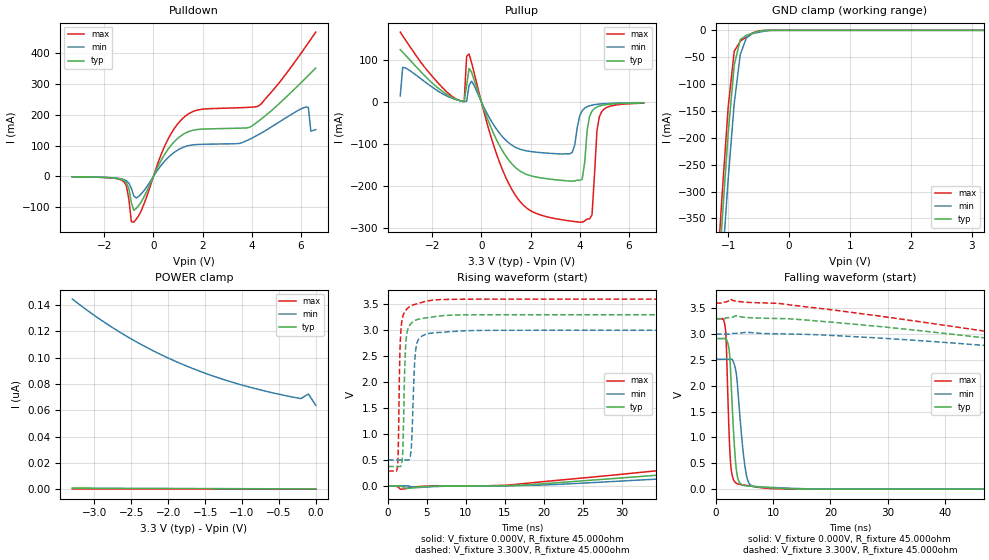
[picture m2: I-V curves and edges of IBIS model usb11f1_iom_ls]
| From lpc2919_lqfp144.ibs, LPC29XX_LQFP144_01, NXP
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| usb11f1
|   Universal Serial Bus Pad
|   Revision 1.1 Specification
|   Programmable Single Ended Core Input
|   Forced Single Ended Low
|   Switchable between
|   - high speed output mode
|   - low speed output mode
|   - low/high speed input mode
| |   Rev 0.20 IBIS Model Design Automation Generation   |
| |   N O N - S I L I C O N   C O R R E L A T E D   |
| |   This IBIS [Model] is pre-Beta tactical support   |
| |  Note: this IBIS [Model] contains clamp curves generated   |
| |   through simulation which should not be relied upon   |
| Pccmos14 hliolib_nlm 4.0
|   0.18 um 3.3V pad library
|   six level metal
|   dual oxide
|   single threshold voltage
|   nominal line mixed supply
|   parasitic extracted netlists
| Process block c14
| Low Speed Output Mode
[Model]   usb11f1_iom_ls | of usb11f1
Model_type   I/O
Polarity   Non-Inverting
Enable   Active-Low
|  Reciever Thresholds
Vinl   = 0.8V
Vinh   = 2.0V
| AC Test Load Conditions
Vref   = 0
Cref   = 0
Rref   = 1000000000
Vmeas   = 1.65
| [Process Range]   typical   min   max
| C_comp edge width   400.000ps   400.000ps   400.000ps
| C_comp Tstrobe   40.000fs   40.000fs   40.000fs
C_comp   3.752pF   3.496pF   4.045pF
[Temperature Range]   25   125   -40
[Voltage Range]   3.30V   3.00V   3.60V
[GND Clamp Reference]   0.00V   0.00V   0.00V
[Pulldown Reference]   0.00V   0.00V   0.00V
[POWER Clamp Reference]   3.30V   3.00V   3.60V
[Pullup Reference]   3.30V   3.00V   3.60V
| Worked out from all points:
|   slope of the pulldown table from 0 to 0.495 V, typ, clamps not added: 6.48 ohm
|   slope of the pullup table from 0 to 0.495 V, typ, clamps not added: 6.61 ohm
|   GND clamp passes 1 mA (typ) near -0.46 V on its own axis
|   rising waveform, V_fixture 0.000V, R_fixture 45.000ohm: 20-80 % time 151ns typ, 180ns min, 132ns max; typ from 0 V to 2.91 V
|   falling waveform, V_fixture 0.000V, R_fixture 45.000ohm: 20-80 % time 850ps typ, 1.23ns min, 609ps max; typ from 2.91 V to 0 V
|   rising waveform, V_fixture 3.300V, R_fixture 45.000ohm: 20-80 % time 318ps typ, 398ps min, 284ps max; typ from 0.374 V to 3.3 V
|   falling waveform, V_fixture 3.300V, R_fixture 45.000ohm: 20-80 % time 156ns typ, 194ns min, 133ns max; typ from 3.3 V to 0.38 V
[GND Clamp]
| ref voltage   0.00V   0.00V   0.00V
|   Voltage   I(typ)   I(min)   I(max)
-3.3V     -4.618A    -4.67A     -4.591A
-1.2V     -533.4mA   -616mA     -486.2mA
-1.1V     -356.1mA   -441.1mA   -306.9mA
-1V       -192.1mA   -277.1mA   -143.8mA
-900mV    -64.59mA   -135.6mA   -38.91mA
-800mV    -17.04mA   -44.51mA   -19.95mA
-700mV    -9.237mA   -13.86mA   -12.52mA
-600mV    -5.456mA   -6.064mA   -4.789mA
-500mV    -1.495mA   -3.666mA   -840.2uA
-300mV    -6.625uA   -179.7uA   -408.9nA
3.2V      293.2pA    68.89nA    105.6pA
[Power Clamp]   | Vtable = Vcc - Vpad
| ref voltage   3.30V   3.00V   3.60V
|   Voltage   I(typ)   I(min)   I(max)
-3.3V     1.005nA    144.5nA    354.7pA
-3V       911.2pA    132nA      335.1pA
-2.6V     800.8pA    117.4nA    309pA
-2.3V     727.5pA    108nA      289.6pA
-1.9V     640.7pA    97.15nA    263.8pA
-1.6V     582.9pA    90.25nA    244.5pA
-1.3V     530.6pA    84.3nA     225.3pA
-1V       483pA      79.18nA    206.1pA
-700mV    439.6pA    74.79nA    187pA
-200mV    377.6pA    68.89nA    155pA
-100mV    416.5pA    72.39nA    142.6pA
0V        319.1pA    63.83nA    125.6pA
[Pulldown]
| ref voltage   0.00V   0.00V   0.00V
|   Voltage   I(typ)   I(min)   I(max)
-3.3V     -1.652mA   -1.454mA   -1.796mA
-1.2V     -13.92mA   -10.45mA   -17.73mA
-1.1V     -21.12mA   -14.45mA   -30.61mA
-900mV    -85.23mA   -38.63mA   -146.6mA
-800mV    -110mA     -63.62mA   -148.7mA
500mV     77.03mA    53.28mA    105.7mA
1.1V      130.5mA    90.36mA    180.9mA
4.3V      181mA      136.8mA    229.8mA
6.2V      319.7mA    225.1mA    421.9mA
6.3V      327.6mA    224.1mA    433.3mA
6.4V      335.5mA    146.8mA    444.9mA
6.6V      351.2mA    151.8mA    468.2mA
[Pullup]   | Vtable = Vcc - Vpad
| ref voltage   3.30V   3.00V   3.60V
|   Voltage   I(typ)   I(min)   I(max)
-3.3V     123.9mA    14.28mA    165.4mA
-3.2V     117.8mA    81.84mA    156.7mA
-800mV    1.807mA    2.206mA    1.368mA
-500mV    79.1mA     39.57mA    113.5mA
1V        -129mA     -91.21mA   -180.1mA
2.5V      -180.9mA   -120.7mA   -269.8mA
3.7V      -188.1mA   -119.1mA   -283mA
4.1V      -182.9mA   -20.96mA   -285.2mA
4.4V      -34.22mA   -9.287mA   -277.5mA
4.5V      -21.68mA   -7.778mA   -267.6mA
4.8V      -9.883mA   -5.195mA   -34.66mA
6.6V      -2.365mA   -1.804mA   -3.161mA
[Ramp]
R_load   = 60.000ohm
|   dV/dt(typ)   dV/dt(min)   dV/dt(max)
dV/dt_r   621.133mV/49.000ns   449.857mV/47.650ns   797.798mV/50.350ns
dV/dt_f   625.100mV/49.850ns   419.096mV/47.300ns   836.278mV/52.000ns
[Rising Waveform]  | cubic spline decimation from 16001 points
V_fixture   = 0.000V
R_fixture   = 45.000ohm
|   Time   V(typ)   V(min)   V(max)
0s        443.9pV    34.49nV    250.2pV
1.75ns    -12.65mV   2.275uV    -62.94mV
15.6ns    5.793mV    2.484mV    18.34mV
130.2ns   1.408V     1.033V     1.795V
182.8ns   2.006V     1.49V      2.541V
215.3ns   2.324V     1.742V     2.891V
240.8ns   2.515V     1.918V     3.033V
308.5ns   2.738V     2.227V     3.184V
402.4ns   2.838V     2.384V     3.248V
800ns     2.907V     2.501V     3.292V
[Falling Waveform]  | cubic spline decimation from 2001 points
V_fixture   = 0.000V
R_fixture   = 45.000ohm
|   Time   V(typ)   V(min)   V(max)
0s        2.914V     2.514V     3.296V
1.65ns    2.918V     2.514V     3.099V
1.8ns     2.902V     2.514V     2.824V
2.25ns    2.726V     2.514V     1.203V
2.75ns    1.81V      2.518V     313.5mV
3.35ns    628.5mV    2.352V     134.1mV
3.85ns    197.5mV    1.878V     99.95mV
5.3ns     62.15mV    280.7mV    75.31mV
6.75ns    52.95mV    48.63mV    46.78mV
100ns     89.79uV    122.2uV    67.53uV
[Rising Waveform]  | cubic spline decimation from 2001 points
V_fixture   = 3.300V
V_fixture_min = 3.000V
V_fixture_max = 3.600V
R_fixture   = 45.000ohm
|   Time   V(typ)   V(min)   V(max)
0s        373.7mV    499.4mV    287.7mV
1.25ns    373.7mV    499.5mV    440.2mV
1.55ns    374.8mV    499.5mV    2.698V
1.85ns    558.6mV    499.5mV    3.237V
2.15ns    2.321V     499.5mV    3.356V
2.4ns     2.919V     499.6mV    3.406V
3ns       3.136V     762.4mV    3.473V
3.6ns     3.197V     2.674V     3.505V
4.85ns    3.237V     2.922V     3.556V
100ns     3.3V       3V         3.6V
[Falling Waveform]  | cubic spline decimation from 16001 points
V_fixture   = 3.300V
V_fixture_min = 3.000V
V_fixture_max = 3.600V
R_fixture   = 45.000ohm
|   Time   V(typ)   V(min)   V(max)
0s        3.3V       3V         3.6V
2.45ns    3.319V     3V         3.678V
28.5ns    3.148V     2.924V     3.35V
114.5ns   2.081V     2.172V     1.981V
188.3ns   1.259V     1.566V     937.8mV
232.7ns   858.8mV    1.248V     557.2mV
289.8ns   591.2mV    921.5mV    405.8mV
389.9ns   453.5mV    659.5mV    332.3mV
557.6ns   398mV      548.8mV    301.5mV
800ns     380mV      513mV      291.2mV
